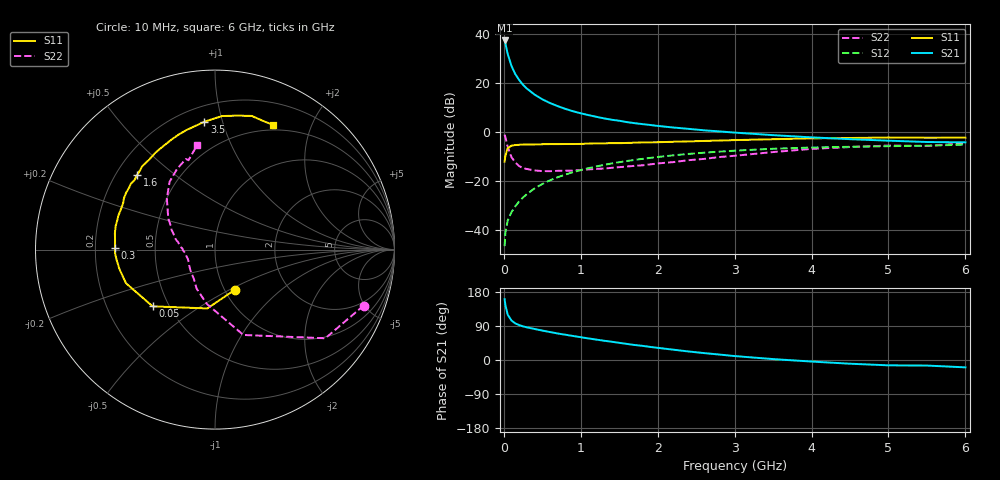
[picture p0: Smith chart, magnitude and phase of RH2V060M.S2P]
! SIEMENS Small Signal Semiconductors
! BFR106
! Si NPN RF Bipolar Junction Transistor in SOT23
! VCE = 2 V  IC = 60 mA
! Common Emitter S-Parameters:  August  1996
# GHz  S  MA  R  50
!  f  S11  S21  S12  S22
! GHz  MAG  ANG  MAG  ANG  MAG  ANG  MAG  ANG
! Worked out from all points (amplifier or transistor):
!   36 points, 10 MHz to 6 GHz, reference 50 ohm
!   highest |S21| = 37.2 dB at 10 MHz (marker M1)
!   |S21| within 3 dB of that: start of sweep to 32.5 MHz
!   unconditionally stable (mu >= 1): 207 MHz to 2.734 GHz; 5.148 GHz to end of sweep
!   at 250 MHz: K = 1.03, MAG = 21.8 dB, |S12| = -26.6 dB
!   at 1.4 GHz: K = 1.06, MAG = 7.4 dB, |S12| = -12.8 dB
!   at 6 GHz: K = 1.01, MAG = -0.1 dB, |S12| = -5.1 dB
!   S11 on the Smith chart (normalised r, x): 10 MHz: 1.12, -0.53; 50 MHz: 0.41, -0.33; 300 MHz: 0.28, +0.01; 1.6 GHz: 0.29, +0.37; 3.5 GHz: 0.30, +0.88; 6 GHz: 0.44, +1.47
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0.01  0.2495 -63.2  72.48 160.5  0.0048 78.1  0.8853 -20.6
0.02  0.3305 -97.4  62.76 145.3  0.009 67.5  0.7885 -38.8
0.05  0.4697 -137.7  38.71 119.7  0.0159 59.9  0.5013 -71.6
0.1  0.5302 -159.3  21.82 104.0  0.0236 62.3  0.3059 -98.6
0.15  0.5435 -168.6  14.91 96.5  0.0311 65.6  0.2399 -115.3
0.2  0.5509 -173.9  11.36 92.1  0.0391 69.1  0.2026 -125.3
0.25  0.5571 -177.7  9.077 88.7  0.0469 70.1  0.1848 -135.1
0.3  0.557 179.1  7.61 86.2  0.0549 71.1  0.1774 -141.3
0.4  0.5593 174.6  5.755 81.8  0.0718 71.7  0.1661 -151.1
0.5  0.5651 170.8  4.625 77.7  0.0878 71.5  0.1609 -157.7
0.6  0.569 166.7  3.879 73.7  0.1046 70.9  0.1603 -161.7
0.7  0.5685 163.4  3.354 70.0  0.1208 69.6  0.1627 -165.5
0.8  0.5706 160.5  2.951 66.7  0.1369 68.1  0.1643 -169.5
1.1  0.583 150.4  2.206 56.9  0.1842 63.8  0.1743 -176.6
1.3  0.5895 144.6  1.898 50.9  0.2147 60.3  0.1812 178.5
1.6  0.6009 136.3  1.591 42.4  0.2578 55.4  0.1993 172.5
2.2  0.6341 121.5  1.236 27.3  0.336 45.2  0.2446 159.8
2.8  0.6715 107.8  1.03 14.4  0.3996 35.1  0.31 146.7
3.5  0.7149 94.7  0.864 2.4  0.4574 24.1  0.3919 133.2
4.5  0.7567 80.5  0.716 -9.8  0.5015 9.9  0.4962 115.3
5.5  0.765 69.2  0.627 -14.7  0.5278 1.3  0.5194 106.5
6  0.7666 65.2  0.617 -19.4  0.5545 -5.5  0.5933 99.5
